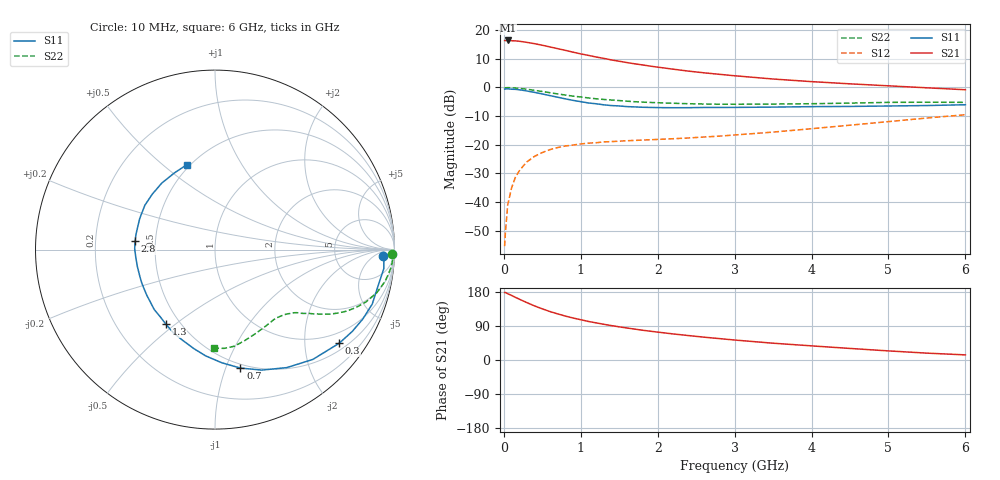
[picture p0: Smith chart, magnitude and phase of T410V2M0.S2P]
! Infineon Technologies  Discrete & RF Semiconductors
! BFR182T
! Si NPN RF Bipolar Junction Transistor in SC75
! VCE = 10 V  IC = 2 mA
! Common Emitter S-Parameters:  October  1999
# GHz  S  MA  R  50
!  f  S11  S21  S12  S22
! GHz  MAG  ANG  MAG  ANG  MAG  ANG  MAG  ANG
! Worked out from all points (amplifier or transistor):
!   36 points, 10 MHz to 6 GHz, reference 50 ohm
!   highest |S21| = 16.4 dB at 50 MHz (marker M1)
!   |S21| within 3 dB of that: start of sweep to 723 MHz
!   unconditionally stable (mu >= 1): 2.089 GHz to 4.49 GHz
!   at 250 MHz: K = 0.15, MSG = 21.7 dB, |S12| = -27.5 dB
!   at 1.4 GHz: K = 0.75, MSG = 14.2 dB, |S12| = -18.9 dB
!   at 6 GHz: K = 0.84, MSG = 4.4 dB, |S12| = -9.5 dB
!   S11 on the Smith chart (normalised r, x): 10 MHz: 22, -13; 300 MHz: 0.68, -2.84; 700 MHz: 0.46, -1.13; 1.3 GHz: 0.42, -0.46; 2.8 GHz: 0.38, +0.04; 6 GHz: 0.48, +0.61
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0.01  0.9348 -2.3  6.587 178.1  0.0017 81.8  0.988 -1.3
0.02  0.9418 -1.3  6.549 178.2  0.0029 96.0  0.9866 -1.0
0.05  0.9464 -6.5  6.604 175.0  0.0089 90.0  0.992 -2.7
0.1  0.931 -12.4  6.531 170.5  0.0176 83.0  0.9877 -5.4
0.15  0.9272 -19.1  6.495 165.4  0.027 78.4  0.9759 -8.0
0.2  0.91 -25.1  6.397 160.6  0.0349 76.4  0.9641 -10.5
0.3  0.8667 -37.0  6.115 151.4  0.0503 70.2  0.9315 -15.1
0.4  0.8195 -48.3  5.804 142.6  0.0629 63.9  0.8905 -19.1
0.5  0.7695 -58.7  5.45 135.0  0.0732 59.1  0.8497 -22.3
0.6  0.72 -68.8  5.089 127.8  0.0823 55.0  0.8089 -25.1
0.7  0.675 -77.9  4.749 121.7  0.0893 51.8  0.7706 -27.3
0.9  0.5946 -95.0  4.125 110.8  0.0989 46.8  0.7049 -30.7
1.1  0.5361 -109.8  3.623 101.7  0.1068 43.8  0.6558 -33.1
1.3  0.4975 -123.4  3.212 94.2  0.1121 42.1  0.6166 -35.2
1.5  0.4756 -135.4  2.865 87.5  0.1155 41.7  0.5901 -36.9
1.8  0.4512 -151.5  2.475 78.6  0.1207 41.5  0.5547 -39.6
2.2  0.4427 -167.4  2.084 68.8  0.1274 43.8  0.5299 -43.2
2.8  0.4478 174.1  1.695 56.5  0.1414 48.3  0.5093 -50.0
3.5  0.4538 157.6  1.403 44.3  0.1663 53.5  0.5128 -58.4
4.5  0.4664 138.5  1.156 30.5  0.2195 57.2  0.533 -71.7
5.5  0.4833 118.0  0.985 18.1  0.2928 56.4  0.5526 -84.7
6  0.4989 108.2  0.912 13.5  0.3343 53.9  0.5492 -90.6
